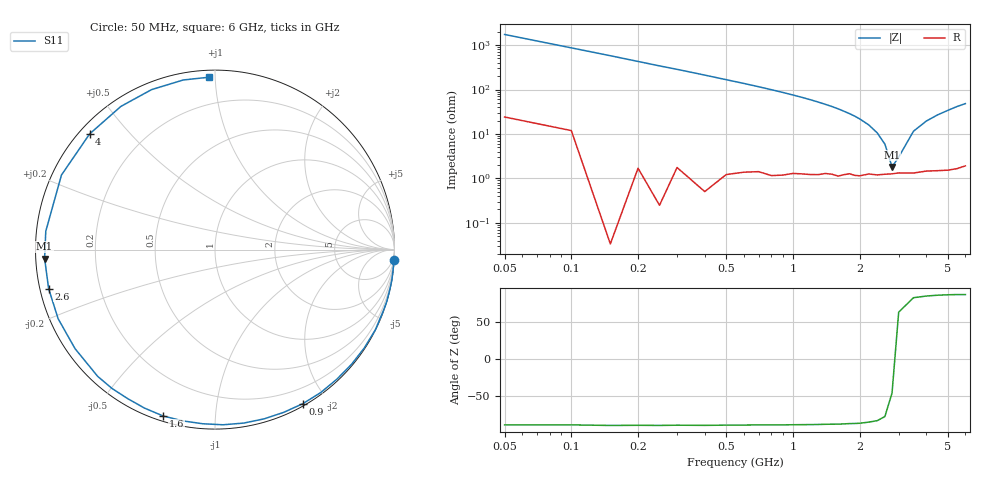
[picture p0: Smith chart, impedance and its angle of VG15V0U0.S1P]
! Infineon Technologies  Discrete & RF Semiconductors
! BB 831
! Si Tuning Diode in SOD323
! VR = 15 V
! S-Parameters:  July  1999
# GHz  S  MA  R  50
!  f  S11
! GHz  MAG  ANG
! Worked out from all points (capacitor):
!   34 points, 50 MHz to 6 GHz, reference 50 ohm
!   read as one part to ground: C = 1.83 pF near 50 MHz
!   lowest |Z| = 1.82 ohm at 2.8 GHz (marker M1)
!   series resonance near 2.865 GHz, so ESL is about 1.7 nH
!   S11 on the Smith chart (normalised r, x): 50 MHz: 0, -35; 900 MHz: 0.02, -1.72; 1.6 GHz: 0.02, -0.74; 2.6 GHz: 0.02, -0.12; 4 GHz: 0.03, +0.39; 6 GHz: 0.04, +0.96
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0.05  0.9992 -3.3
0.15  1 -9.9
0.25  0.9998 -16.7
0.4  0.9989 -26.6
0.6  0.9936 -40.0
0.8  0.9907 -53.5
0.9  0.9881 -60.3
1  0.9843 -67.1
1.1  0.9819 -73.8
1.2  0.9798 -80.6
1.3  0.977 -87.4
1.4  0.9727 -94.1
1.6  0.9711 -107.3
1.7  0.9664 -114.0
1.8  0.9624 -120.3
1.9  0.9632 -126.5
2  0.9623 -132.8
2.2  0.9553 -144.7
2.4  0.9551 -156.2
2.6  0.9521 -166.8
2.8  0.9506 -177.0
3  0.9483 173.8
3.5  0.951 154.1
4  0.9505 137.3
4.5  0.9547 123.3
5  0.9589 111.6
5.5  0.9614 100.6
6  0.9611 92.0
